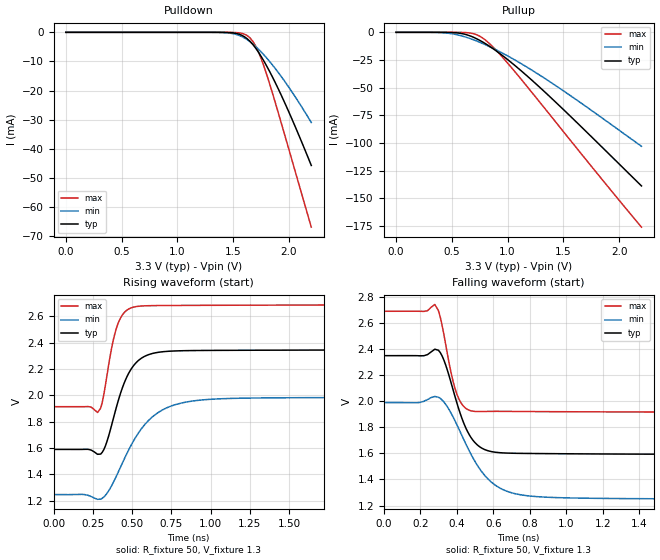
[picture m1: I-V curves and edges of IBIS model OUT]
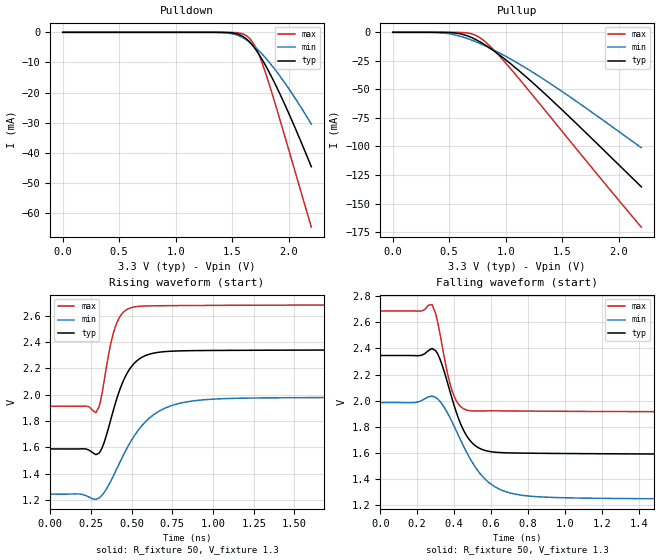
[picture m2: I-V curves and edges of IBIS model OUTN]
|   IBIS File of SG2520EGN C
|   LV-PECL, Vcc=3.3V, fo<=212.5MHz
[IBIS Ver]   3.2
[File Name]   sg2520egn_33v.ibs
[File Rev]   1.0
[Date]   Sep. 2, 2020
[Source]
[Notes]
Created by Minoru Kozaki
[Disclaimer]
Seiko Epson Corporation makes no warranty with respect to the
information contained herein.
[Copyright]
Copyright(C) 2020, Seiko Epson Corporation. All rights reserved.
|   Component
[Component]   SG2520EGN
[Manufacturer]  Seiko Epson Corporation
[Package]
R_pkg   17.7m   NA   NA
L_pkg   235p   NA   NA
C_pkg   208f   NA   NA
[Pin]   signal_name   model_name   R_pin   L_pin   C_pin
1   OE/ST   NC
2   NC   NC
3   GND   GND
4   OUT   OUT   17.7m   235p   208f
5   OUTN   OUTN   10.4m   129p   221f
6   VCC   POWER
[Diff Pin] inv_pin  vdiff  tdelay_typ
4   5   0   0
| Models and submodels in the file (2): OUT (Output_ECL), OUTN (Output_ECL)
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|   Model OUT
[Model]   OUT
Model_type   Output_ECL
Polarity   Non-Inverting
Vref = 1.3
Vmeas = 1.966
Rref = 50
Cref = 0
C_comp   0.5p   0.5p   0.5p
[Temperature Range]   25   105   -40
[Voltage Range]   3.3   2.97   3.63
[Pullup Reference]   3.3   2.97   3.63
[Pulldown Reference]   3.3   2.97   3.63
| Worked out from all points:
|   falling waveform, R_fixture 50, V_fixture 1.3: 20-80 % time 112ps typ, 184ps min, 71ps max; typ from 2.35 V to 1.59 V
|   rising waveform, R_fixture 50, V_fixture 1.3: 20-80 % time 130ps typ, 230ps min, 78.4ps max; typ from 1.59 V to 2.35 V
[Pullup]
0V        25.96nA    13.28nA    125.7nA
400mV     -16.71uA   -275.2uA   -2.782uA
550mV     -548.3uA   -2.249mA   -27.26uA
625mV     -1.952mA   -4.308mA   -238.1uA
700mV     -4.719mA   -6.95mA    -1.407mA
750mV     -7.237mA   -8.967mA   -3.49mA
800mV     -10.17mA   -11.16mA   -6.889mA
875mV     -15.16mA   -14.72mA   -13.84mA
975mV     -22.63mA   -19.92mA   -24.86mA
1.275V    -48.51mA   -37.87mA   -61.5mA
1.625V    -81.97mA   -61.6mA    -105.4mA
2.2V      -138.9mA   -103.1mA   -176.2mA
[Pulldown]
0V        25.96nA    13.28nA    125.7nA
1.4V      -18.52uA   -75.52uA   -3.777uA
1.525V    -362.7uA   -703.8uA   -77.58uA
1.625V    -2.191mA   -2.503mA   -1.099mA
1.675V    -4.133mA   -3.952mA   -3.028mA
1.7V      -5.36mA    -4.797mA   -4.598mA
1.725V    -6.734mA   -5.711mA   -6.585mA
1.775V    -9.847mA   -7.722mA   -11.59mA
1.85V     -15.2mA    -11.12mA   -20.63mA
1.95V     -23.2mA    -16.2mA    -33.68mA
2.075V    -34.12mA   -23.27mA   -50.32mA
2.2V      -45.74mA   -30.98mA   -66.93mA
[Falling Waveform]
R_fixture = 50
V_fixture = 1.3
V_fixture_min = 0.97
V_fixture_max = 1.63
0s        2.349V     1.989V     2.69V
220ps     2.349V     1.999V     2.689V
280ps     2.399V     2.037V     2.742V
300ps     2.391V     2.03V      2.695V
330ps     2.315V     1.994V     2.51V
400ps     1.992V     1.823V     2.059V
490ps     1.699V     1.563V     1.923V
630ps     1.606V     1.339V     1.922V
860ps     1.598V     1.266V     1.92V
4ns       1.59V      1.247V     1.914V
[Rising Waveform]
R_fixture = 50
V_fixture = 1.3
V_fixture_min = 0.97
V_fixture_max = 1.63
0s        1.589V     1.246V     1.913V
280ps     1.552V     1.21V      1.869V
300ps     1.553V     1.212V     1.901V
330ps     1.614V     1.24V      2.073V
370ps     1.773V     1.313V     2.358V
410ps     1.949V     1.411V     2.541V
530ps     2.252V     1.694V     2.673V
700ps     2.331V     1.892V     2.681V
980ps     2.34V      1.968V     2.682V
4ns       2.348V     1.988V     2.689V
[Ramp]
R_load = 50
dV/dt_r   0.45340/129.71p   0.44316/229.15p   0.46331/77.78p
dV/dt_f   0.45340/111.19p   0.44316/182.79p   0.46331/70.44p
|   Model OUTN
[Model]   OUTN
Model_type   Output_ECL
Polarity   Inverting
Vref = 1.3
Vmeas = 1.966
Rref = 50
Cref = 0
C_comp   0.5p   0.5p   0.5p
[Temperature Range]   25   105   -40
[Voltage Range]   3.3   2.97   3.63
[Pullup Reference]   3.3   2.97   3.63
[Pulldown Reference]   3.3   2.97   3.63
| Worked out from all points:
|   falling waveform, R_fixture 50, V_fixture 1.3: 20-80 % time 112ps typ, 184ps min, 70.5ps max; typ from 2.35 V to 1.59 V
|   rising waveform, R_fixture 50, V_fixture 1.3: 20-80 % time 131ps typ, 232ps min, 78.4ps max; typ from 1.59 V to 2.34 V
[Pullup]
0V        27.87nA    13.28nA    125.7nA
400mV     -16.71uA   -274.9uA   -2.782uA
550mV     -546.8uA   -2.236mA   -27.25uA
625mV     -1.938mA   -4.273mA   -237.7uA
700mV     -4.664mA   -6.881mA   -1.397mA
750mV     -7.136mA   -8.87mA    -3.441mA
800mV     -10.01mA   -11.03mA   -6.749mA
875mV     -14.88mA   -14.53mA   -13.48mA
975mV     -22.18mA   -19.64mA   -24.13mA
1.275V    -47.37mA   -37.24mA   -59.53mA
1.625V    -79.9mA    -60.47mA   -102mA
2.2V      -135.4mA   -101.1mA   -170.7mA
[Pulldown]
0V        25.96nA    13.28nA    125.7nA
1.4V      -18.52uA   -75.49uA   -3.777uA
1.525V    -362uA     -701.9uA   -77.54uA
1.625V    -2.174mA   -2.487mA   -1.092mA
1.675V    -4.085mA   -3.92mA    -2.987mA
1.7V      -5.289mA   -4.754mA   -4.515mA
1.725V    -6.635mA   -5.656mA   -6.44mA
1.775V    -9.681mA   -7.639mA   -11.27mA
1.85V     -14.91mA   -10.98mA   -19.97mA
1.95V     -22.7mA    -15.98mA   -32.56mA
2.075V    -33.34mA   -22.92mA   -48.62mA
2.2V      -44.63mA   -30.48mA   -64.68mA
[Falling Waveform]
R_fixture = 50
V_fixture = 1.3
V_fixture_min = 0.97
V_fixture_max = 1.63
0s        2.345V     1.986V     2.685V
220ps     2.346V     1.999V     2.684V
280ps     2.399V     2.035V     2.735V
320ps     2.329V     2V         2.534V
390ps     2.008V     1.833V     2.071V
430ps     1.84V      1.713V     1.962V
480ps     1.706V     1.573V     1.925V
620ps     1.607V     1.343V     1.923V
840ps     1.598V     1.268V     1.92V
4ns       1.589V     1.247V     1.913V
[Rising Waveform]
R_fixture = 50
V_fixture = 1.3
V_fixture_min = 0.97
V_fixture_max = 1.63
0s        1.588V     1.245V     1.912V
280ps     1.544V     1.206V     1.863V
320ps     1.602V     1.24V      2.024V
370ps     1.803V     1.34V      2.377V
400ps     1.935V     1.415V     2.516V
450ps     2.108V     1.543V     2.626V
520ps     2.243V     1.694V     2.666V
700ps     2.326V     1.895V     2.675V
980ps     2.335V     1.964V     2.677V
4ns       2.343V     1.984V     2.684V
[Ramp]
R_load = 50
dV/dt_r   0.45146/130.30p   0.44139/230.60p   0.46121/77.69p
dV/dt_f   0.45146/111.16p   0.44139/183.19p   0.46121/70.06p
